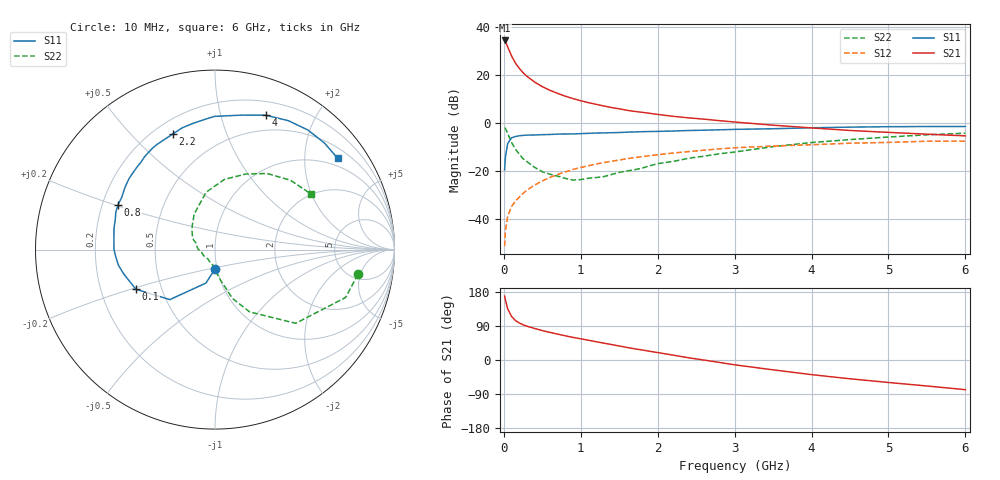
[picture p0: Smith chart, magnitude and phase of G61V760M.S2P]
! SIEMENS Small Signal Semiconductors
! BFG193
! Si NPN RF Bipolar Junction Transistor in SOT223
! VCE = 1.75 V  IC = 60 mA
! Common Emitter S-Parameters:  August  1996
# GHz  S  MA  R  50
!  f  S11  S21  S12  S22
! GHz  MAG  ANG  MAG  ANG  MAG  ANG  MAG  ANG
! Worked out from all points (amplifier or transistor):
!   36 points, 10 MHz to 6 GHz, reference 50 ohm
!   highest |S21| = 34.5 dB at 10 MHz (marker M1)
!   |S21| within 3 dB of that: start of sweep to 54.42 MHz
!   unconditionally stable (mu >= 1): start of sweep to 12.32 MHz; 247 MHz to 2.752 GHz
!   at 250 MHz: K = 1.00, MAG = 24.9 dB, |S12| = -29.3 dB
!   at 1.4 GHz: K = 1.09, MAG = 9.4 dB, |S12| = -15.9 dB
!   at 6 GHz: K = 0.97, MSG = 1.1 dB, |S12| = -7.5 dB
!   S11 on the Smith chart (normalised r, x): 10 MHz: 0.98, -0.21; 100 MHz: 0.36, -0.21; 800 MHz: 0.27, +0.21; 2.2 GHz: 0.27, +0.66; 4 GHz: 0.33, +1.39; 6 GHz: 0.76, +2.83
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0.01  0.106 -89.3  53.35 168.7  0.0027 79.1  0.8081 -9.8
0.02  0.193 -105.1  50.43 158.8  0.0055 71.9  0.7754 -20.1
0.05  0.3756 -132.1  39.24 135.0  0.0115 65.9  0.6089 -42.4
0.1  0.4931 -153.4  25.46 115.2  0.0182 64.0  0.3972 -60.9
0.15  0.5263 -165.1  18.05 104.1  0.0235 64.3  0.2874 -70.5
0.2  0.5453 -170.9  14.01 97.9  0.0284 66.4  0.2256 -74.1
0.25  0.5551 -176.2  11.31 93.0  0.0341 67.2  0.1811 -78.7
0.3  0.5629 179.9  9.531 89.2  0.04 68.0  0.1573 -81.9
0.4  0.5668 173.4  7.213 83.3  0.051 68.3  0.1194 -87.7
0.5  0.5751 168.0  5.789 77.6  0.0621 67.5  0.0968 -93.0
0.6  0.5803 163.2  4.85 72.9  0.0738 66.2  0.0859 -99.1
0.8  0.5953 155.1  3.653 63.8  0.0961 62.7  0.0703 -118.5
1.1  0.6128 144.0  2.679 52.1  0.129 57.1  0.0707 -148.5
1.3  0.6259 137.0  2.281 44.4  0.1504 52.8  0.0765 -169.4
1.6  0.6491 127.3  1.858 33.2  0.181 45.6  0.1004 171.6
2.2  0.6854 110.2  1.391 12.9  0.2378 31.3  0.159 143.1
2.8  0.7265 94.9  1.129 -6.3  0.2906 16.7  0.229 120.6
3.5  0.7644 78.6  0.907 -26.0  0.3328 -1.1  0.3238 98.7
4  0.8003 69.3  0.796 -38.6  0.3544 -11.1  0.3943 82.4
4.5  0.8263 60.4  0.704 -49.6  0.3817 -21.3  0.454 68.0
5.5  0.851 44.3  0.589 -68.6  0.4195 -44.4  0.5715 42.5
6  0.8522 36.7  0.543 -78.3  0.4203 -57.5  0.6179 30.1
